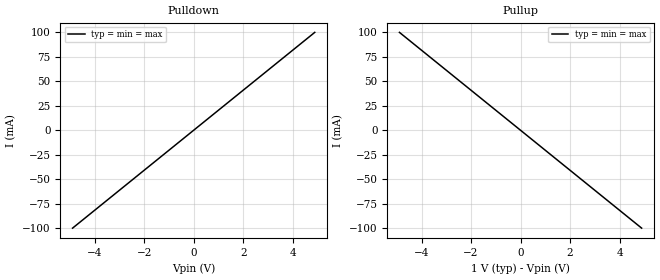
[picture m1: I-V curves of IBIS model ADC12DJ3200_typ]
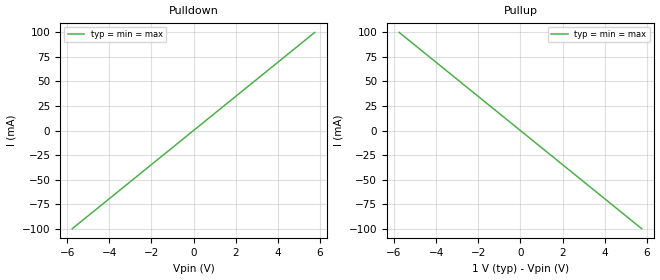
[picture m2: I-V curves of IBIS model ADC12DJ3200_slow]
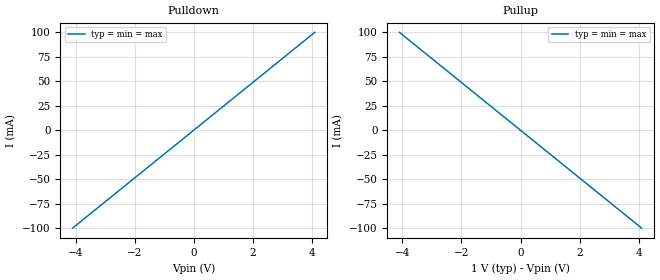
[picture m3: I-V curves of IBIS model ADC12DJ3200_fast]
[IBIS Ver] 6.0
[File Name]  ADC12DJ3200.ibs
[File Rev]   1.1
[Source]   Developed by: John Baprawski; John Baprawski Inc.; www.serdesdesign.com
[Notes]   v1.0   initial version, May 2021
   v1.1   reduced slope on Ramp statement, since this triggered memory warning in HyperLynx, 2/14/2022
[Component]   ADC12DJ3200
[Manufacturer] Texas Instruments Deutschland GmbH
[Pin]   signal_name   model_name   R_pin L_pin  C_pin
2p   ADC12DJ3200_2p   ADC12DJ3200
2n   ADC12DJ3200_2n   ADC12DJ3200
[Diff_Pin] inv_pin vdiff tdelay_typ tdelay_min tdelay_max
2p   2n   NA   NA   NA   NA
[Package]
R_pkg  0.0   0.0   0.0
L_pkg  0.0   0.0   0.0
C_pkg  0.0   0.0   0.0
[Model Selector] ADC12DJ3200
ADC12DJ3200_typ   typical
ADC12DJ3200_slow   slow
ADC12DJ3200_fast   fast
ADC12DJ3200_leakage   leakage
ADC12DJ3200_tempinv   tempinv
| Models and submodels in the file (5): ADC12DJ3200_typ (Output), ADC12DJ3200_slow (Output), ADC12DJ3200_fast (Output), ADC12DJ3200_leakage (Output), ADC12DJ3200_tempinv (Output)
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[Model] ADC12DJ3200_typ
Model_type Output
C_comp   0   0   0
Cref = 0
Vref = 0.5
Rref = 50
Vmeas = 0.5
[Temperature_Range] 25 125 0
[Voltage Range]  1  1  1
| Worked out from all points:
|   slope of the pulldown table from 0 to 0.15 V, typ, clamps not added: 48.9 ohm
|   slope of the pullup table from 0 to 0.15 V, typ, clamps not added: 48.9 ohm
[Pulldown]
-4.893V   -100mA     -100mA     -100mA
0V        0A         0A         0A
4.893V    100mA      100mA      100mA
[Pullup]
-4.893V   100mA      100mA      100mA
0V        0A         0A         0A
4.893V    -100mA     -100mA     -100mA
[Ramp]
dV/dt_r 0.2/1p 0.2/1p 0.2/1p
dV/dt_f 0.2/1p 0.2/1p 0.2/1p
[Algorithmic Model]
Executable Windows_cl19.00.24215.1_64 ADC12DJ3200_x64.dll ADC12DJ3200_typ.ami
Executable Linux_gcc4.7.4_64 ADC12DJ3200_x64.so ADC12DJ3200_typ.ami
[End Algorithmic Model]
[Model] ADC12DJ3200_slow
Model_type Output
C_comp   0   0   0
Cref = 0
Vref = 0.5
Rref = 50
Vmeas = 0.5
[Temperature_Range] 25 125 0
[Voltage Range]  1  1  1
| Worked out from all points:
|   slope of the pulldown table from 0 to 0.15 V, typ, clamps not added: 57.6 ohm
|   slope of the pullup table from 0 to 0.15 V, typ, clamps not added: 57.6 ohm
[Pulldown]
-5.757V   -100mA     -100mA     -100mA
0V        0A         0A         0A
5.757V    100mA      100mA      100mA
[Pullup]
-5.757V   100mA      100mA      100mA
0V        0A         0A         0A
5.757V    -100mA     -100mA     -100mA
[Ramp]
dV/dt_r 0.2/1p 0.2/1p 0.2/1p
dV/dt_f 0.2/1p 0.2/1p 0.2/1p
[Algorithmic Model]
Executable Windows_cl19.00.24215.1_64 ADC12DJ3200_x64.dll ADC12DJ3200_slow.ami
Executable Linux_gcc4.7.4_64 ADC12DJ3200_x64.so ADC12DJ3200_slow.ami
[End Algorithmic Model]
[Model] ADC12DJ3200_fast
Model_type Output
C_comp   0   0   0
Cref = 0
Vref = 0.5
Rref = 50
Vmeas = 0.5
[Temperature_Range] 25 125 0
[Voltage Range]  1  1  1
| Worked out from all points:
|   slope of the pulldown table from 0 to 0.15 V, typ, clamps not added: 41 ohm
|   slope of the pullup table from 0 to 0.15 V, typ, clamps not added: 41 ohm
[Pulldown]
-4.101V   -100mA     -100mA     -100mA
0V        0A         0A         0A
4.101V    100mA      100mA      100mA
[Pullup]
-4.101V   100mA      100mA      100mA
0V        0A         0A         0A
4.101V    -100mA     -100mA     -100mA
[Ramp]
dV/dt_r 0.2/1p 0.2/1p 0.2/1p
dV/dt_f 0.2/1p 0.2/1p 0.2/1p
[Algorithmic Model]
Executable Windows_cl19.00.24215.1_64 ADC12DJ3200_x64.dll ADC12DJ3200_fast.ami
Executable Linux_gcc4.7.4_64 ADC12DJ3200_x64.so ADC12DJ3200_fast.ami
[End Algorithmic Model]
